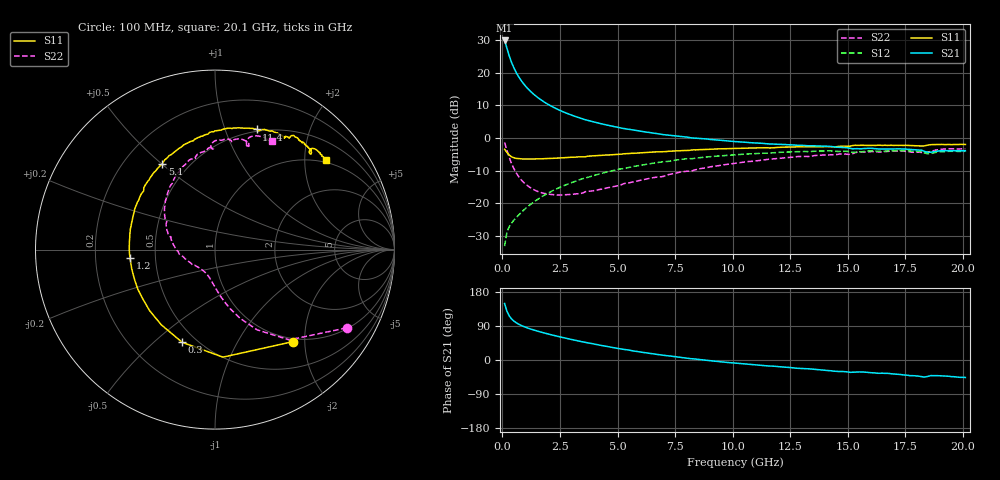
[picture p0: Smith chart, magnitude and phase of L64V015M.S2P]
!  Infineon Technologies AG
! BFR380L3 , PF131585-7, No.6, Th 09.10.01, soldered on pcb-board, measured with PP GSG850
!  Vce=4.0 V,  Ic=15.0 mA
! Common Emitter S-Parameters:  15. November 2001
#  GHz  S  MA  R  50
! f  S11  S21  S12  S22
! GHz  Mag  Ang  Mag  Ang  Mag  Ang  Mag  Ang
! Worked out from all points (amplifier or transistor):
!   201 points, 100 MHz to 20.1 GHz, reference 50 ohm
!   highest |S21| = 29.9 dB at 100 MHz (marker M1)
!   |S21| within 3 dB of that: start of sweep to 225.2 MHz
!   unconditionally stable (mu >= 1): 1.62 GHz to 4.413 GHz
!   at 3.4 GHz: K = 1.02, MAG = 8.5 dB, |S12| = -12.7 dB
!   at 10.1 GHz: K = 0.95, MSG = 2.0 dB, |S12| = -5.2 dB
!   at 20.1 GHz: K = 0.99, MSG = 0.1 dB, |S12| = -4.1 dB
!   S11 on the Smith chart (normalised r, x): 100 MHz: 0.94, -1.76; 300 MHz: 0.42, -0.62; 1.2 GHz: 0.36, -0.04; 5.1 GHz: 0.36, +0.50; 11.4 GHz: 0.48, +1.29; 20.1 GHz: 0.93, +2.53
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0.1  0.6727 -49.6  31.18 149.0  0.02201 67.2  0.8532 -30.8
0.2  0.6007 -85.8  23.61 128.6  0.03591 57.5  0.6511 -50.6
0.3  0.5481 -109.5  18.09 116.5  0.04373 52.9  0.5042 -62.4
0.4  0.5149 -125.5  14.43 108.5  0.04947 52.1  0.4062 -70.1
0.5  0.4984 -137.0  11.92 102.8  0.05489 52.8  0.3402 -75.6
0.6  0.4872 -145.6  10.11 98.5  0.06038 54.1  0.2936 -79.9
0.7  0.4833 -152.8  8.788 94.9  0.06555 55.3  0.2593 -83.5
0.8  0.4789 -158.4  7.754 91.7  0.07123 56.5  0.2334 -86.5
0.9  0.4766 -163.2  6.934 89.1  0.07689 57.5  0.213 -89.3
1  0.4762 -167.4  6.278 86.7  0.08273 58.4  0.1975 -91.9
1.2  0.4758 -174.5  5.276 82.3  0.09445 59.6  0.1747 -96.7
1.6  0.4792 174.7  4.012 74.9  0.1192 60.8  0.1491 -105.5
2  0.4854 166.2  3.25 68.4  0.1441 60.7  0.1379 -113.9
2.6  0.4967 155.2  2.55 59.7  0.1819 59.1  0.1342 -126.3
3.5  0.5144 141.3  1.954 47.7  0.2385 55.0  0.1436 -142.2
5.1  0.5618 121.4  1.436 29.6  0.3347 45.5  0.1882 -169.8
6.8  0.6148 103.8  1.154 13.9  0.4244 34.5  0.254 165.1
10.1  0.692 78.8  0.8804 -8.1  0.5524 13.0  0.4096 130.3
11.4  0.7081 70.9  0.8224 -15.1  0.5855 4.6  0.4645 118.2
13.5  0.7339 61.0  0.7605 -24.2  0.6248 -8.0  0.5326 101.3
16.8  0.7716 48.4  0.6795 -35.6  0.6325 -24.3  0.6261 79.2
20.1  0.7955 38.9  0.6374 -46.1  0.6264 -38.2  0.6842 62.5
